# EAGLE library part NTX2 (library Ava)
Radiometrix NTX2 Transmitter Module Author Anthony Stirk / http://ava.upuaut.net
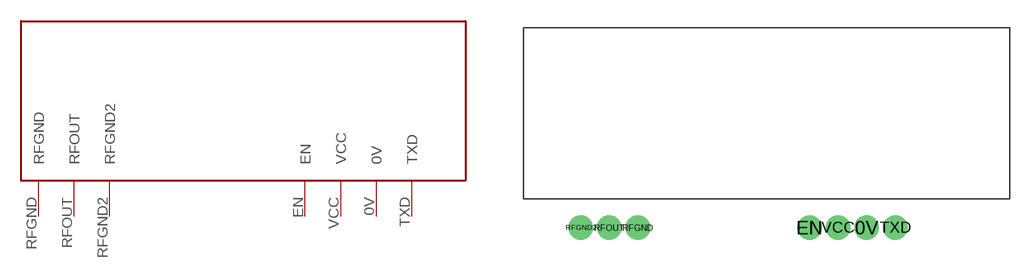
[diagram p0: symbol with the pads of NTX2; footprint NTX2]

Designator prefix -

## NTX2  [NTX2]
0V  0V
EN  EN
RFGND  RFGND
RFGND2  RFGND2
RFOUT  RFOUT
TXD  TXD
VCC  VCC

## Footprint NTX2 (pad centres in mm)
Radiometrix NTX2 http://www.radiometrix.com/files/additional/ntx2nrx2.pdf Flat mounted orientation
drill 0.7 pad 2.184: 0V -2.54,-10.16; EN -7.62,-10.16; RFGND -22.86,-10.16; RFGND2 -27.94,-10.16; RFOUT -25.4,-10.16; TXD 0,-10.16; VCC -5.08,-10.16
